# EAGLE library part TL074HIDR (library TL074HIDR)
Quad, 40-V, 5-MHz, 4-mV offset voltage, 20-V/s, In to V+ op amp with -40C to 125C operation Source: Datasheet
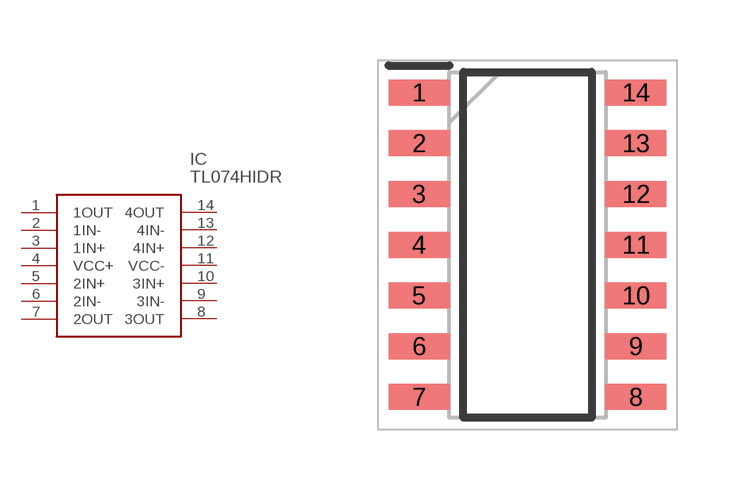
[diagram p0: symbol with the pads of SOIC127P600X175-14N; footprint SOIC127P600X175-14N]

Designator prefix IC

## TL074HIDR (Arrow_Part_Number: TL074HIDR; Arrow_Price-Stock: null?utm_currency=USD&region=nac; Description: Quad, 40-V, 5-MHz, 4-mV offset voltage, 20-V/s, In to V+ op amp with -40C to 125C operation; Height: 1.75mm; Manufacturer_Name: Texas Instruments; Manufacturer_Part_Number: TL074HIDR; Mouser_Part_Number: 595-TL074HIDR; Mouser_Price-Stock: https://www.mouser.co.uk/ProductDetail/Texas-Instruments/TL074HIDR?qs=81r%252BiQLm7BSo1sbhfEy0IA%3D%3D)  [SOIC127P600X175-14N]
1  1OUT
2  1IN-
3  1IN+
4  VCC+
5  2IN+
6  2IN-
7  2OUT
8  3OUT
9  3IN-
10  3IN+
11  VCC-
12  4IN+
13  4IN-
14  4OUT

## Footprint SOIC127P600X175-14N (pad centres in mm)
D (-R-PDSO-G14)
smd 1.525 x 0.65: 1 -2.712,3.81; 2 -2.712,2.54; 3 -2.712,1.27; 4 -2.712,0; 5 -2.712,-1.27; 6 -2.712,-2.54; 7 -2.712,-3.81; 8 2.712,-3.81; 9 2.712,-2.54; 10 2.712,-1.27; 11 2.712,0; 12 2.712,1.27; 13 2.712,2.54; 14 2.712,3.81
